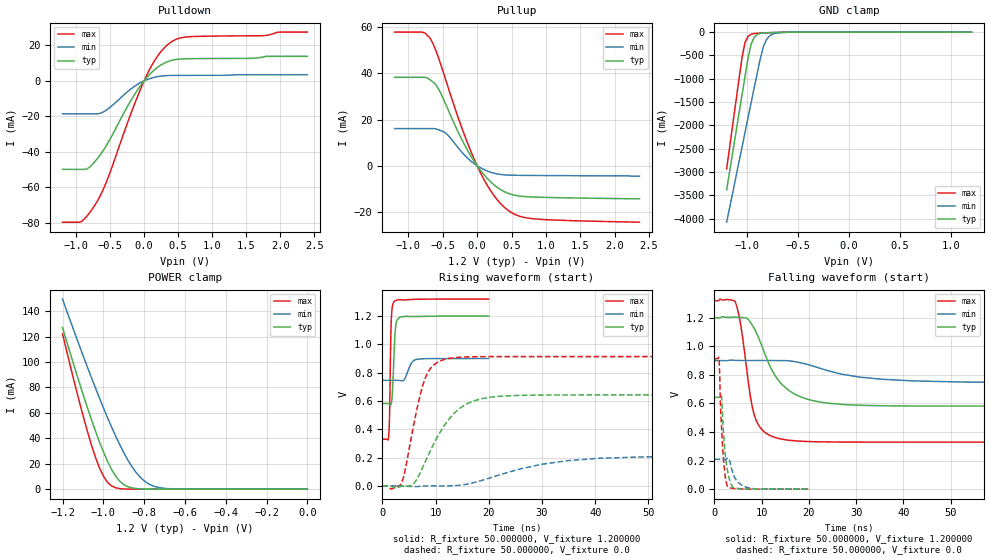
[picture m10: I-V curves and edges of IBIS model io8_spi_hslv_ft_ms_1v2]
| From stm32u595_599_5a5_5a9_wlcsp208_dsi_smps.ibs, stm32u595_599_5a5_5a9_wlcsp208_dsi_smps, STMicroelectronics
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|   Model io8_spi_hslv_ft_ms_1v2
[Model]  io8_spi_hslv_ft_ms_1v2
Model_type I/O
Polarity   Non-Inverting
Enable   Active-Low
Vinl =   0.360000V
Vinh =   0.840000V
Vmeas =  0.600000V
Cref =   50.000000pF
Rref =   100.000000M
Vref =   0.0V
C_comp   3.133100pF   3.070300pF   3.178200pF
[Temperature Range]   25.000000   0.140000k   -40.000000
[Pullup Reference]   1.200000V   0.900000V   1.320000V
[Pulldown Reference]   0.0V   0.0V   0.0V
[POWER Clamp Reference]   1.200000V   0.900000V   1.320000V
[GND Clamp Reference]   0.0V   0.0V   0.0V
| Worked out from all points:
|   slope of the pulldown table from 0 to 0.18 V, typ, clamps not added: 25.4 ohm
|   slope of the pullup table from 0 to 0.18 V, typ, clamps not added: 27.8 ohm
|   GND clamp passes 1 mA (typ) near -0.51 V on its own axis
|   POWER clamp passes 1 mA (typ) near -0.86 V on its own axis
|   rising waveform, R_fixture 50.000000, V_fixture 1.200000: 20-80 % time 439ps typ, 1.02ns min, 262ps max; typ from 0.582 V to 1.2 V
|   rising waveform, R_fixture 50.000000, V_fixture 0.0: 20-80 % time 5.96ns typ, 13.8ns min, 3.13ns max; typ from 0 V to 0.643 V
|   falling waveform, R_fixture 50.000000, V_fixture 1.200000: 20-80 % time 6.09ns typ, 13.1ns min, 2.67ns max; typ from 1.2 V to 0.582 V
|   falling waveform, R_fixture 50.000000, V_fixture 0.0: 20-80 % time 1.05ns typ, 1.79ns min, 828ps max; typ from 0.643 V to 0 V
[Pulldown]
|Voltage   I(typ)   I(min)   I(max)
-1.2V     -49.85mA   -18.57mA   -79.56mA
-920mV    -49.85mA   -18.57mA   -79.19mA
-840mV    -49.59mA   -18.57mA   -76.08mA
-720mV    -45.32mA   -18.57mA   -69.74mA
-560mV    -36.71mA   -16.58mA   -57.44mA
-200mV    -11.43mA   -4.739mA   -19.03mA
0V        0A         -500fA     0A
160mV     6.476mA    2.075mA    11.78mA
360mV     10.99mA    2.989mA    20.81mA
480mV     12.07mA    3.053mA    23.52mA
640mV     12.43mA    3.074mA    24.76mA
2.4V      13.78mA    3.432mA    27.43mA
[Pullup]
|Voltage   I(typ)   I(min)   I(max)
-1.2V     38.32mA    16.09mA    57.93mA
-800mV    38.32mA    16.09mA    57.93mA
-680mV    37.18mA    16.09mA    55.12mA
-560mV    33.2mA     15.59mA    46.69mA
-440mV    25.53mA    13.72mA    35.67mA
-200mV    10.05mA    5.175mA    14.59mA
0V        580fA      234pA      0A
200mV     -7.072mA   -2.851mA   -11mA
440mV     -11.84mA   -4.03mA    -19.1mA
600mV     -13.07mA   -4.154mA   -21.71mA
840mV     -13.59mA   -4.223mA   -23.04mA
2.36V     -14.3mA    -4.5mA     -24.47mA
[GND_clamp]
|Voltage   I(typ)   I(min)   I(max)
-1.2V     -3.379A    -4.076A    -2.932A
-1.05V    -1.35A     -2.47A     -550.7mA
-1.02V    -947.8mA   -2.149A    -221.5mA
-990mV    -552.4mA   -1.829A    -88.44mA
-960mV    -255.3mA   -1.51A     -44.87mA
-930mV    -111.8mA   -1.191A    -30.68mA
-870mV    -28.35mA   -564.6mA   -21.34mA
-840mV    -18.65mA   -309.5mA   -18.49mA
-810mV    -14.07mA   -161.6mA   -15.92mA
-780mV    -11.37mA   -83.33mA   -13.53mA
-600mV    -3.009mA   -4.321mA   -3.091mA
1.2V      0A         13.65nA    0A
[POWER_clamp]
|Voltage   I(typ)   I(min)   I(max)
-1.2V     127mA      149.4mA    122.2mA
-1.12V    84.97mA    114mA      70.27mA
-1.06V    55.51mA    88.42mA    35.67mA
-1.02V    37.63mA    72.04mA    17.17mA
-1V       29.51mA    64.13mA    10.3mA
-960mV    15.69mA    48.99mA    2.571mA
-900mV    3.624mA    28.77mA    182.8uA
-840mV    490.7uA    13.24mA    11.35uA
-800mV    116.8uA    6.532mA    1.77uA
-740mV    13.2uA     1.723mA    109.1nA
-620mV    167.4nA    79.36uA    0A
0V        0A         17.87nA    0A
[Ramp]
| variable   typ   min   max
dV/dt_r  0.38564/5.95494n   0.12553/13.81090n   0.54826/3.11360n
dV/dt_f  0.37079/6.08385n   92.43600m/13.08890n 0.59435/2.66116n
R_load = 50.000000
[Rising Waveform]
R_fixture= 50.000000
V_fixture= 1.200000
V_fixture_min= 0.900000
V_fixture_max= 1.320000
|time   V(typ)   V(min)   V(max)
0s        582mV      746mV      329.4mV
1.201ns   582.1mV    746mV      359.5mV
1.361ns   580.2mV    746mV      510.8mV
1.562ns   573.9mV    746mV      1.006V
1.682ns   579.3mV    746mV      1.177V
2.202ns   937.1mV    746mV      1.301V
2.563ns   1.142V     746.1mV    1.31V
3.283ns   1.191V     745mV      1.316V
6.326ns   1.197V     892.9mV    1.318V
19.94ns   1.2V       900mV      1.32V
[Rising Waveform]
R_fixture= 50.000000
V_fixture= 0.0
V_fixture_min= 0.0
V_fixture_max= 0.0
|time   V(typ)   V(min)   V(max)
0s        1.999nV    239.3nV    1.184nV
3.604ns   -2.104mV   -33.41uV   18.96mV
6.006ns   20.73mV    -5.305mV   452.6mV
8.008ns   165.7mV    -726.8uV   756.7mV
10.01ns   322.4mV    -291.1uV   864.5mV
13.21ns   502.8mV    1.105mV    904.7mV
20.82ns   628.5mV    63.82mV    913.4mV
34.83ns   642.3mV    178.2mV    913.7mV
48.45ns   642.6mV    204.3mV    913.7mV
199.4ns   642.7mV    209.3mV    913.8mV
[Falling Waveform]
R_fixture= 50.000000
V_fixture= 1.200000
V_fixture_min= 0.900000
V_fixture_max= 1.320000
|time   V(typ)   V(min)   V(max)
0s        1.2V       900mV      1.32V
4.404ns   1.205V     902.1mV    1.313V
5.606ns   1.202V     901.1mV    1.141V
7.608ns   1.169V     901.1mV    649.5mV
8.809ns   1.1V       901.2mV    483.8mV
12.01ns   843.8mV    901mV      372.4mV
15.22ns   705.9mV    899.9mV    345mV
23.22ns   605.9mV    837.7mV    331.2mV
42.44ns   582.6mV    757.9mV    329.4mV
199.4ns   582mV      746mV      329.4mV
[Falling Waveform]
R_fixture= 50.000000
V_fixture= 0.0
V_fixture_min= 0.0
V_fixture_max= 0.0
|time   V(typ)   V(min)   V(max)
0s        642.7mV    209.3mV    913.8mV
961ps     642.8mV    209.3mV    918.1mV
1.321ns   652.4mV    209.4mV    547.6mV
1.481ns   651.6mV    209.4mV    450.9mV
1.802ns   457.5mV    209.4mV    261.3mV
2.322ns   232.7mV    209.3mV    82mV
2.803ns   122.7mV    216.7mV    19.79mV
3.884ns   14.65mV    114mV      5.679mV
6.446ns   2.129mV    17.68mV    1.23mV
19.94ns   1.999nV    239.3nV    1.184nV
